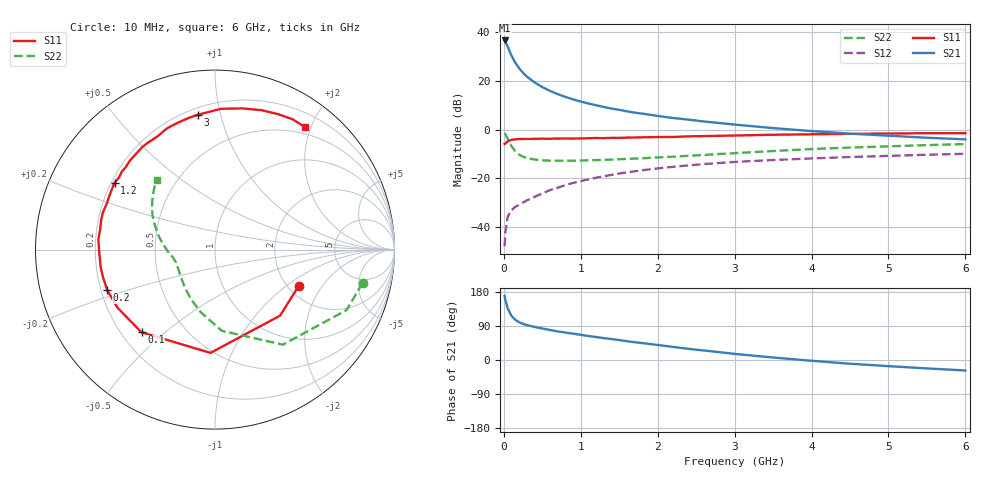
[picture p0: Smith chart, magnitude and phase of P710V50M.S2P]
! SIEMENS Small Signal Semiconductors
! BFP196
! Si NPN RF Bipolar Junction Transistor in SOT143
! VCE = 10 V  IC = 50 mA
! Common Emitter S-Parameters:  May  1996
# GHz  S  MA  R  50
!  f  S11  S21  S12  S22
! GHz  MAG  ANG  MAG  ANG  MAG  ANG  MAG  ANG
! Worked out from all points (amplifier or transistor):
!   36 points, 10 MHz to 6 GHz, reference 50 ohm
!   highest |S21| = 36.7 dB at 10 MHz (marker M1)
!   |S21| within 3 dB of that: start of sweep to 55.95 MHz
!   unconditionally stable (mu >= 1): 532 MHz to 4.649 GHz
!   at 250 MHz: K = 0.77, MSG = 26.7 dB, |S12| = -30.0 dB
!   at 1.4 GHz: K = 1.09, MAG = 11.9 dB, |S12| = -18.6 dB
!   at 6 GHz: K = 0.98, MSG = 3.0 dB, |S12| = -9.9 dB
!   S11 on the Smith chart (normalised r, x): 10 MHz: 2.26, -1.25; 100 MHz: 0.28, -0.42; 200 MHz: 0.23, -0.17; 1.2 GHz: 0.21, +0.29; 3 GHz: 0.24, +0.85; 6 GHz: 0.40, +1.91
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0.01  0.5081 -23.7  68.47 169.1  0.004 72.4  0.8428 -12.8
0.02  0.5167 -45.4  64.34 158.6  0.0078 69.6  0.8068 -24.7
0.05  0.576 -92.5  50.99 136.3  0.0162 54.4  0.6508 -54.5
0.1  0.6163 -131.6  33.28 116.1  0.0221 45.8  0.4541 -85.2
0.15  0.6323 -149.2  23.67 105.8  0.0259 45.7  0.3565 -103.2
0.2  0.6412 -159.4  18.29 99.5  0.0285 47.6  0.3066 -115.8
0.25  0.6428 -166.0  14.71 95.2  0.0316 50.0  0.2769 -125.4
0.3  0.6443 -171.3  12.34 92.1  0.0351 51.5  0.261 -132.0
0.4  0.6457 -179.4  9.379 87.2  0.0414 55.4  0.2424 -142.3
0.5  0.652 175.2  7.508 83.2  0.0488 57.5  0.2337 -149.1
0.6  0.6497 170.1  6.27 79.2  0.0569 58.7  0.2305 -153.7
0.7  0.6551 165.4  5.396 75.4  0.0637 59.4  0.2294 -157.3
0.9  0.6549 157.6  4.197 69.5  0.0799 58.9  0.2294 -162.8
1.1  0.665 150.2  3.454 63.4  0.095 57.6  0.234 -166.4
1.2  0.6725 146.3  3.171 60.6  0.1025 57.1  0.2366 -168.1
1.6  0.6856 133.9  2.38 49.6  0.1318 52.2  0.2501 -173.7
2.2  0.7073 117.1  1.736 34.6  0.172 43.9  0.2772 177.7
3  0.757 97.4  1.271 16.1  0.2164 32.5  0.3279 165.2
3.5  0.7855 87.5  1.077 6.6  0.2372 25.7  0.3632 157.6
4.5  0.8189 71.5  0.827 -9.8  0.2731 14.0  0.4278 145.1
5.5  0.8451 59.2  0.681 -22.2  0.3043 3.6  0.4805 134.9
6  0.8468 53.6  0.631 -27.7  0.3189 -2.0  0.5052 130.0
